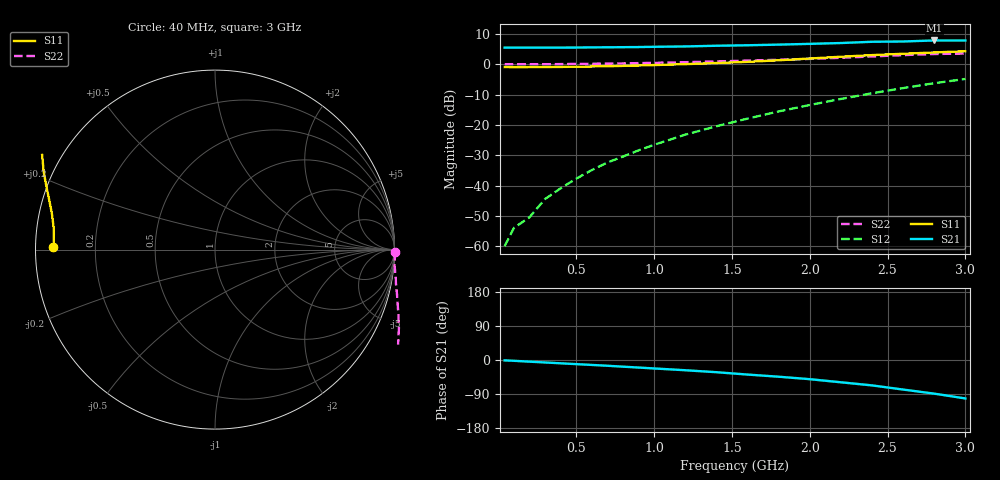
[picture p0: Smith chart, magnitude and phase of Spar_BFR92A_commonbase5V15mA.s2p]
! Filename:  BFR92ACD.S2P  Version:  2.0
! NXP part #: BFR92A  Date: Jul 1990
! Bias condition: Vce=5V, Ic=15mA
! COMMON BASE
#  MHz  S  MA  R  50
! Freq  S11  S21  S12  S22
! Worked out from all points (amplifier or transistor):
!   21 points, 40 MHz to 3 GHz, reference 50 ohm
!   highest |S21| = 7.9 dB at 2.8 GHz (marker M1)
!   |S21| within 3 dB of that: start of sweep to end of sweep
!   unconditionally stable (mu >= 1): nowhere
!   at 300 MHz: K = -0.60, MSG = 25.0 dB, |S12| = -44.4 dB
!   at 1 GHz: K = -0.95, MSG = 16.2 dB, |S12| = -26.6 dB
!   at 3 GHz: K = -0.89, MSG = 6.3 dB, |S12| = -4.8 dB
40  0.901 179.2  1.885 -1.0  0.001 40.6  1.002 -0.7
100  0.899 178.0  1.883 -2.1  0.002 88.4  1.004 -1.4
200  0.9 176.3  1.882 -4.4  0.003 112.7  1.003 -3.0
300  0.902 174.5  1.881 -6.5  0.006 124.6  1.003 -4.6
400  0.905 172.9  1.885 -8.7  0.009 132.8  1.008 -6.1
500  0.912 171.1  1.89 -10.9  0.013 137.6  1.014 -7.6
600  0.92 169.5  1.902 -13.0  0.018 142.2  1.02 -9.1
700  0.929 167.8  1.908 -15.2  0.024 144.3  1.026 -10.7
800  0.942 166.0  1.916 -17.6  0.03 145.8  1.035 -12.3
900  0.955 164.4  1.925 -19.9  0.038 147.4  1.046 -14.1
1000  0.971 162.6  1.943 -22.3  0.047 148.2  1.056 -15.7
1200  1.006 159.2  1.97 -27.0  0.069 148.8  1.083 -19.4
1400  1.049 155.5  2.023 -32.2  0.095 147.3  1.114 -23.1
1600  1.098 151.3  2.06 -38.4  0.127 146.4  1.149 -27.4
1800  1.165 147.2  2.111 -44.1  0.167 143.8  1.187 -32.3
2000  1.246 142.9  2.173 -50.6  0.213 140.8  1.227 -38.0
2200  1.333 138.3  2.243 -58.8  0.268 137.2  1.28 -44.8
2400  1.418 133.0  2.352 -67.0  0.333 132.4  1.347 -52.4
2600  1.492 126.1  2.378 -78.0  0.405 127.2  1.418 -60.6
2800  1.568 117.6  2.473 -88.8  0.488 120.2  1.478 -69.2
3000  1.643 108.2  2.468 -101.5  0.573 113.1  1.504 -78.8
